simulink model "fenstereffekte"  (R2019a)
settings: Solver=ode45  StartTime=0.0  StopTime=10.0  RelTol=1e-3  EnableMultiTasking=on
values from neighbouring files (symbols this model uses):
  ampl = 10    [fenstereffekte_3.m]    (also in leakage_1.m)
  fsig = 100.5    [fenstereffekte_3.m]
  N = 1024    [fenstereffekte_3.m]    (also in leakage_1.m = 20; fenster_funkt_2.m; psd_noise_4.m)
  phi = pi/3    (= 1.0471975512)    [fenstereffekte_3.m]    (also in leakage_1.m)
  pw = sum(hanning(N).^2)/N    [fenstereffekte_3.m]    (also in psd_noise_4.m)
  Ts = 1/fs    (= 0.0009765625)    [fenstereffekte_3.m]    (also in leakage_1.m = 0.05; psd_noise_4.m)
libraries: dspspect3 x2, dspsigops x2

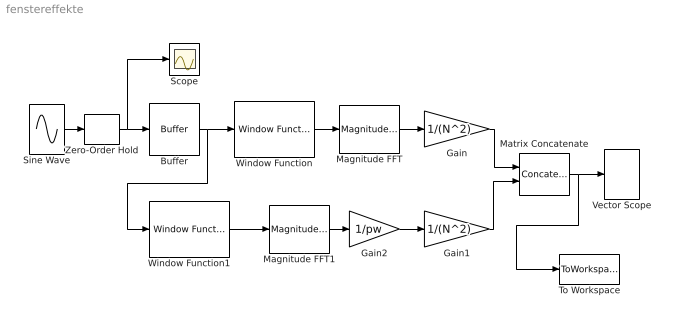
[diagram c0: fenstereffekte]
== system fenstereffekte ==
  Buffer : Buffer  N=N
  Gain : Gain  Gain=1/(N^2)
  Gain1 : Gain  Gain=1/(N^2)
  Gain2 : Gain  Gain=1/pw
  Magnitude FFT : dspspect3/Magnitude FFT  mag_or_magsq=Magnitude squared  FFTImplementation=Auto  fftLenInherit=on  fftsize=256  WrapInput=on
  Magnitude FFT1 : dspspect3/Magnitude FFT  mag_or_magsq=Magnitude squared  FFTImplementation=Auto  fftLenInherit=on  fftsize=256  WrapInput=on
  Matrix Concatenate : Concatenate  Mode=Multidimensional array  ConcatenateDimension=2
  Scope : Scope
  Sine Wave : Sin  Amplitude=ampl  Frequency=2*pi*fsig  Phase=phi  SampleTime=0
  To Workspace : ToWorkspace  VariableName=Y  SampleTime=-1
  Vector Scope : SpectrumAnalyzer
  Window Function : dspsigops/Window Function  winmode=Apply window to input  wintype=Boxcar  sampmode=Continuous  samptime=1  N=64  Rs=50  beta=10  winsamp=Symmetric  UserWindow=fenster  OptParams=on  UserParams={'symmetric'}  dataType=double  isSigned=on  wordLen=16  udDataType=sfix(16)  fracBitsMode=Best precision  numFracBits=15  roundingMode=Floor  overflowMode=off  numSidelobes=4  sidelobeLevel=-30
  Window Function1 : dspsigops/Window Function  winmode=Apply window to input  wintype=Hanning  sampmode=Continuous  samptime=1  N=64  Rs=50  beta=10  winsamp=Symmetric  UserWindow=fenster  OptParams=on  UserParams={'symmetric'}  dataType=double  isSigned=on  wordLen=16  udDataType=sfix(16)  fracBitsMode=Best precision  numFracBits=15  roundingMode=Floor  overflowMode=off  numSidelobes=4  sidelobeLevel=-30
  Zero-Order Hold : ZeroOrderHold  SampleTime=Ts
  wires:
  Sine Wave/1 -> Zero-Order Hold/1
  Zero-Order Hold/1 -> Scope/1, Buffer/1
  Buffer/1 -> Window Function1/1, Window Function/1
  Magnitude FFT/1 -> Gain/1
  Window Function/1 -> Magnitude FFT/1
  Magnitude FFT1/1 -> Gain2/1
  Gain1/1 -> Matrix Concatenate/2
  Window Function1/1 -> Magnitude FFT1/1
  Gain/1 -> Matrix Concatenate/1
  Matrix Concatenate/1 -> To Workspace/1, Vector Scope/1
  Gain2/1 -> Gain1/1
